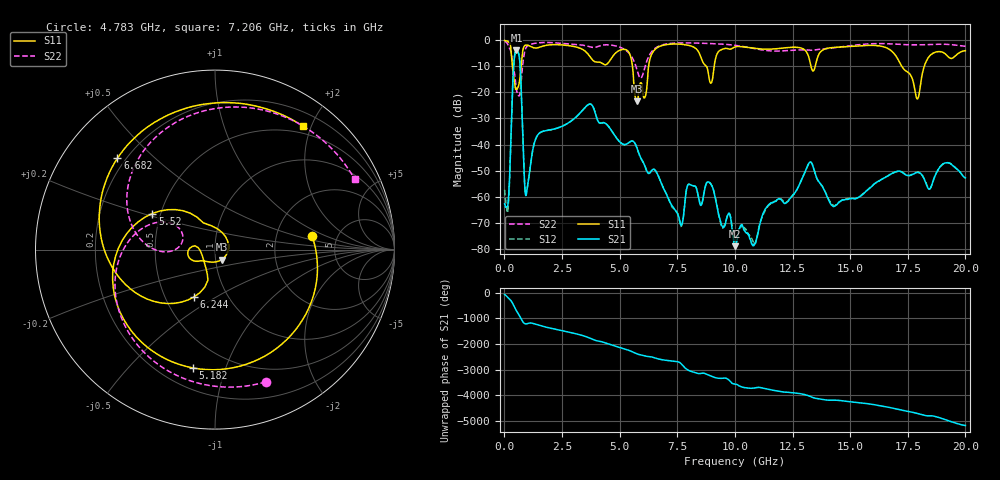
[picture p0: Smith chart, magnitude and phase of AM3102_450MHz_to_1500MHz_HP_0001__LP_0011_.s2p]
!Agilent Technologies,E8364B,MY43040894,A.07.50.67
!Agilent E8364B: A.07.50.67
!Date: Thursday, January 11, 2018 05:20:14
!Correction: S11(Full 2 Port(1,2))
!S21(Full 2 Port(1,2))
!S12(Full 2 Port(1,2))
!S22(Full 2 Port(1,2))
!S2P File: Measurements: S11, S21, S12, S22:
# Hz S  dB  R 50
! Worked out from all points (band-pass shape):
!   1601 points, 10 MHz to 20 GHz, reference 50 ohm
!   highest |S21| = -3.87 dB at 522.2 MHz (marker M1); lowest = -79.0 dB at 10.02 GHz (marker M2)
!   |S21| within 3 dB of the highest: 431.4 MHz to 654.7 MHz (223.3 MHz wide, 41.1 % of centre)
!   lowest |S11| = -23.5 dB at 5.745 GHz (marker M3), VSWR 1.14, Z = 53.5 - j5.98 ohm
!   |S11| at or under -10 dB: 347.7 MHz to 726.1 MHz (378.4 MHz wide, 70.5 % of centre); 5.556 GHz to 6.256 GHz (699.4 MHz wide, 11.8 % of centre); 17.24 GHz to 18.21 GHz (971.8 MHz wide, 5.48 % of centre)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
!   |S22| runs from -21.3 to -0.4 dB; largest |S21 - S12| = 0.0018
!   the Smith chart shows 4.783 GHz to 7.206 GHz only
!   S11 on the Smith chart (normalised r, x): 4.783 GHz: 3.23, +0.72; 5.182 GHz: 0.32, -0.78; 5.52 GHz: 0.45, +0.22; 6.244 GHz: 0.70, -0.40; 6.682 GHz: 0.17, +0.39; 7.206 GHz: 0.39, +1.87
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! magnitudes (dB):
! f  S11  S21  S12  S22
! 10 MHz  -0.1  -62.7  -57.4  -0.4
! 172.4 MHz  -0.6  -61.2  -63.5  -2.2
! 522.2 MHz  -18.7  -3.9  -3.9  -19.0
! 959.5 MHz  -1.8  -58.8  -58.6  -2.6
! 1.459 GHz  -2.8  -36.2  -36.2  -1.0
! 3.346 GHz  -3.3  -27.3  -27.3  -1.8
! 4.783 GHz  -5.3  -36.5  -36.5  -2.1
! 5.182 GHz  -3.5  -40.0  -40.0  -3.3
! 5.52 GHz  -7.9  -38.7  -38.7  -6.2
! 5.745 GHz  -23.5  -41.1  -41.2  -11.1
! 6.244 GHz  -10.8  -51.1  -51.1  -6.5
! 6.682 GHz  -2.6  -52.1  -52.1  -2.3
! 7.206 GHz  -1.5  -62.5  -62.6  -1.2
! 8.893 GHz  -15.2  -54.6  -54.5  -1.2
! 10.01 GHz  -2.5  -78.6  -77.6  -1.9
! 10.02 GHz  -2.5  -79.0  -77.5  -1.9
! 13.34 GHz  -11.1  -47.3  -47.3  -3.8
! 14.27 GHz  -2.8  -63.8  -63.3  -2.9
! 16.68 GHz  -3.3  -51.8  -51.9  -1.3
! 17.91 GHz  -22.5  -50.7  -50.6  -1.7
! 18.5 GHz  -5.6  -56.5  -56.5  -1.6
! 20 GHz  -4.0  -52.8  -52.8  -2.3
